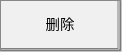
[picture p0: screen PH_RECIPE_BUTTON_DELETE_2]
VISUALIZATION PH_RECIPE_BUTTON_DELETE_2  // 122x52
VAR_IN_OUT
	RECIPE_CTRL_V2 : ST_RecipeCtrl_2;
END_VAR
    Button (0,0 120x50), "删除", input disabled if: (RECIPE_CTRL_V2.sStatus.bBusy) <> 0, text list: 'TextList_Recipe', text index: 114
        p55702900: SEL(RECIPE_CTRL_V2.sCmd.bRecipeDel, 16#000000, 16#00FF00)
        tap RECIPE_CTRL_V2.sCmd.bRecipeDel
END_VISUALIZATION
